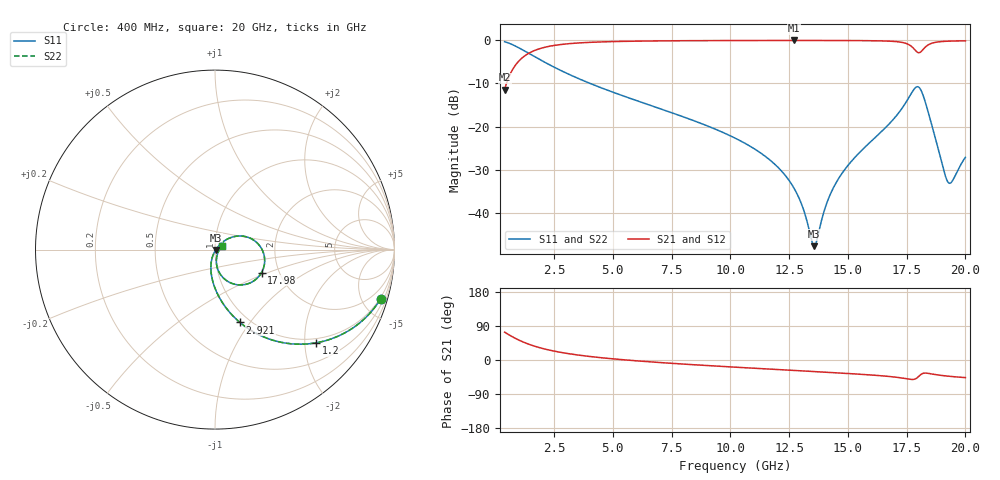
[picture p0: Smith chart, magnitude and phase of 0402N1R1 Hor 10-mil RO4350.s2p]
# GHz S MA R 50
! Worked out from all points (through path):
!   1960 points, 400 MHz to 20 GHz, reference 50 ohm
!   highest |S21| = -0.04 dB at 12.7 GHz (marker M1); lowest = -11.4 dB at 400 MHz (marker M2)
!   group delay of S21, straight-line fit = 12.6 ps
!   lowest |S11| = -47.8 dB at 13.57 GHz (marker M3), VSWR 1.01, Z = 50.3 - j0.226 ohm
!   |S11| at or under -10 dB: 4.034 GHz to end of sweep
!   |S22| runs from -47.8 to -0.3 dB; largest |S21 - S12| = 0
!   S11 on the Smith chart (normalised r, x): 400 MHz: 0.90, -6.79; 1.2 GHz: 0.90, -2.25; 2.921 GHz: 0.90, -0.90; 17.98 GHz: 1.62, -0.45; 20 GHz: 1.08, +0.04
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0.4  0.9633 -16.5  0.2683 73.5  0.2683 73.5  0.9633 -16.5
1.200408  0.7654 -42.8  0.6428 47.2  0.6428 47.2  0.7654 -42.8
1.980807  0.581 -58.9  0.8127 31.0  0.8127 31.0  0.581 -58.9
2.921286  0.4293 -71.1  0.9016 18.7  0.9016 18.7  0.4293 -71.1
3.671669  0.3475 -77.8  0.9359 11.9  0.9359 11.9  0.3475 -77.8
6.943338  0.1634 -95.6  0.9839 -6.4  0.9839 -6.4  0.1634 -95.6
10.205  0.0733 -106.6  0.9938 -18.9  0.9938 -18.9  0.0733 -106.6
11.72578  0.04004 -109.3  0.9953 -24.2  0.9953 -24.2  0.04004 -109.3
12.69627  0.01955 -106.6  0.9956 -27.5  0.9956 -27.5  0.01955 -106.6
13.09648  0.01125 -98.8  0.9955 -28.9  0.9955 -28.9  0.01125 -98.8
13.46667  0.00471 -61.1  0.9954 -30.1  0.9954 -30.1  0.00471 -61.1
13.56672  0.004095 -33.2  0.9953 -30.5  0.9953 -30.5  0.004095 -33.2
14.127  0.01344 38.2  0.9949 -32.4  0.9949 -32.4  0.01344 38.2
14.60725  0.02493 44.5  0.9942 -34.2  0.9942 -34.2  0.02493 44.5
16.73834  0.1059 38.1  0.9779 -43.3  0.9779 -43.3  0.1059 38.1
17.57876  0.2129 16.2  0.8952 -50.3  0.8952 -50.3  0.2129 16.2
17.97897  0.2892 -26.2  0.7215 -45.3  0.7215 -45.3  0.2892 -26.2
18.16907  0.2428 -54.2  0.7658 -35.9  0.7658 -35.9  0.2428 -54.2
18.44921  0.137 -78.4  0.8944 -35.5  0.8944 -35.5  0.137 -78.4
19.24962  0.02285 -40.5  0.9764 -42.6  0.9764 -42.6  0.02285 -40.5
19.42971  0.02301 -9.3  0.9801 -43.7  0.9801 -43.7  0.02301 -9.3
20  0.04386 26.7  0.9857 -46.5  0.9857 -46.5  0.04386 26.7
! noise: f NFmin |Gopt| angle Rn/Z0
0.4  0.00135  0.8243  5.407  0.00161
2.571  0.005087  0.6823  8.227  0.003086
4.752  0.008072  0.6382  12.49  0.004161
6.933  0.01077  0.6119  16.98  0.005042
9.104  0.01334  0.5951  21.47  0.005853
11.29  0.01599  0.5868  25.93  0.006737
13.47  0.01925  0.5931  30.31  0.008124
15.64  0.02662  0.6501  34.66  0.01323
17.82  0.1611  0.9241  39.52  0.4167
20  0.04023  0.7023  43.93  0.0229
